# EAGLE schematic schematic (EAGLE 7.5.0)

## Sheet 1 of 3: Supply
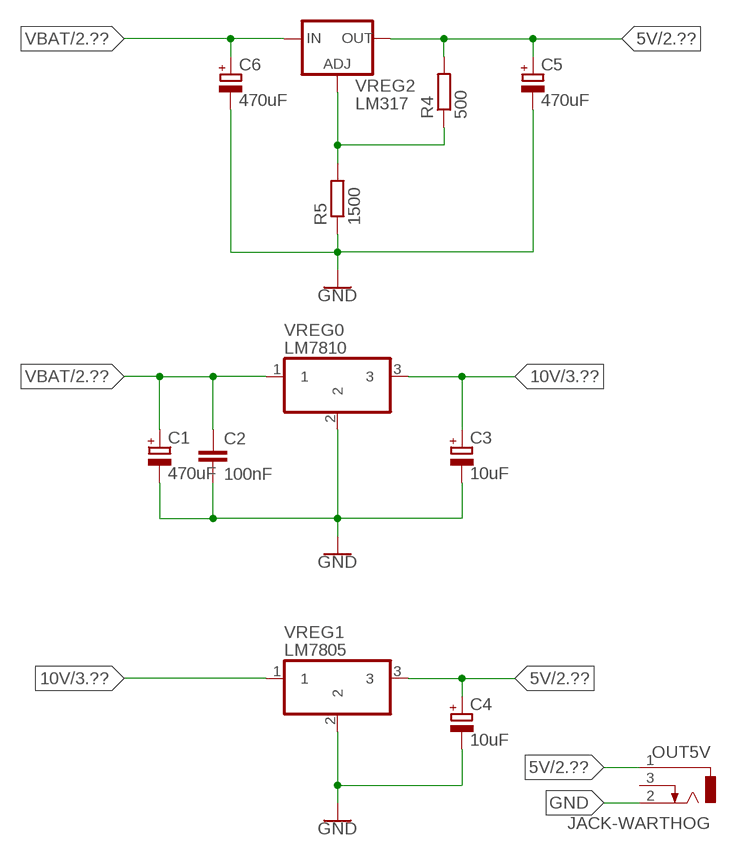
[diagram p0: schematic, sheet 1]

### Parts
C1  470uF  CPOL-EUE3.5-8  [E3,5-8]
C2  100nF  C-EUC0805  [C0805]
C3  10uF  CPOL-EUSMCC  [SMC_C]
C4  10uF  CPOL-EUSMCC  [SMC_C]
C5  470uF  CPOL-EUSMCC  [SMC_C]
C6  470uF  CPOL-EUSMCC  [SMC_C]
OUT5V  JACK-WARTHOG  [JACK-WARTHOG]
R4  500  R-EU_R0805  [R0805]
R5  1500  R-EU_R0805  [R0805]
VREG0  LM7810  TO220V-WARTHOG  [TO220V-WARTHOG]
VREG1  LM7805  TO220V-WARTHOG  [TO220V-WARTHOG]
VREG2  LM317  V_REG_317DPACK  [V-REG_DPACK]

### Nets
5V: C4.+ C5.+ OUT5V.1 R4.2 VREG1.3 VREG2.4(OUT) ; also sheet 2,3
10V: C3.+ VREG0.3 VREG1.1 ; also sheet 3
ADJ: R4.1 R5.2 VREG2.1(ADJ)
GND: C1.- C2.2 C3.- C4.- C5.- C6.- OUT5V.2 R5.1 VREG0.2 VREG1.2 ; also sheet 2,3
VBAT: C1.+ C2.1 C6.+ VREG0.1 VREG2.3(IN) ; also sheet 2,3
Unconnected: OUT5V.3

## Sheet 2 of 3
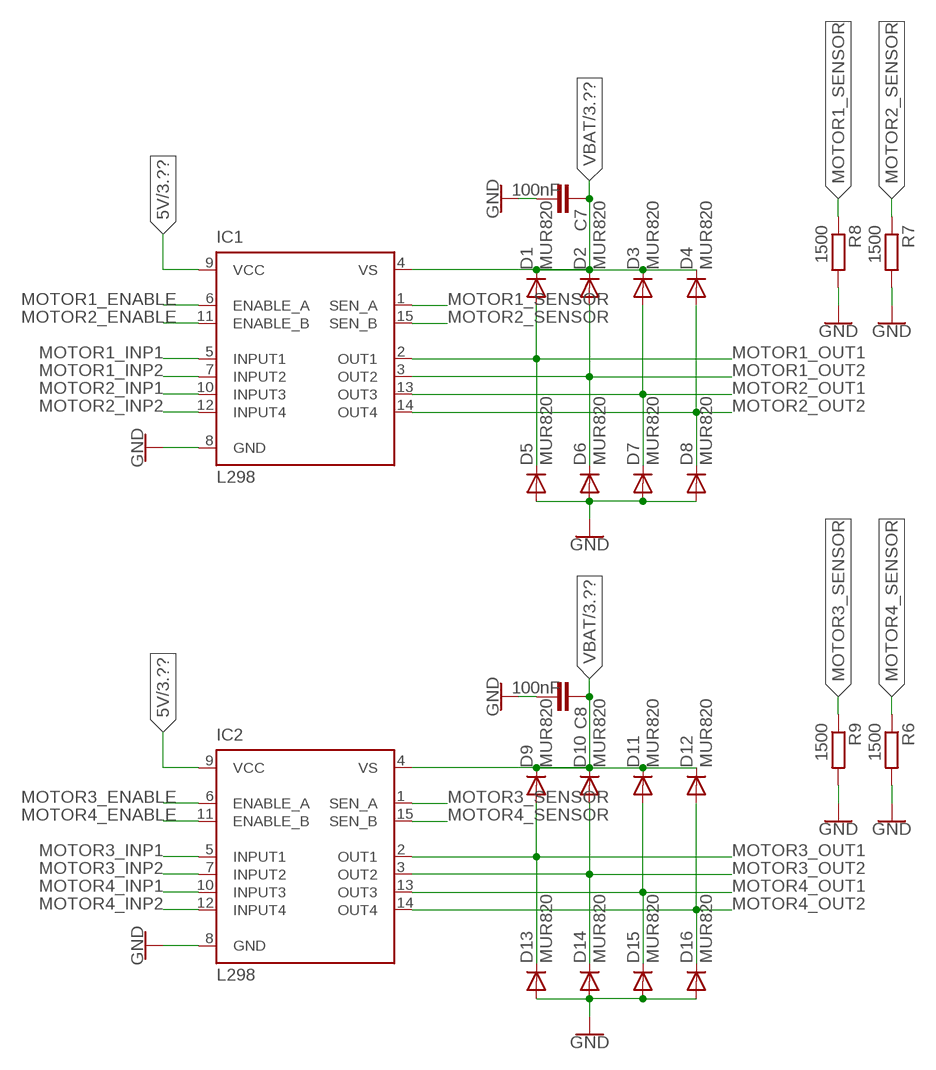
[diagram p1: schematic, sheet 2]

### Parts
C7  100nF  C-EUC0805  [C0805]
C8  100nF  C-EUC0805  [C0805]
D1  MUR820  [C221B1A]
D2  MUR820  [C221B1A]
D3  MUR820  [C221B1A]
D4  MUR820  [C221B1A]
D5  MUR820  [C221B1A]
D6  MUR820  [C221B1A]
D7  MUR820  [C221B1A]
D8  MUR820  [C221B1A]
D9  MUR820  [C221B1A]
D10  MUR820  [C221B1A]
D11  MUR820  [C221B1A]
D12  MUR820  [C221B1A]
D13  MUR820  [C221B1A]
D14  MUR820  [C221B1A]
D15  MUR820  [C221B1A]
D16  MUR820  [C221B1A]
IC1  L298  [MULTIWATT-15]
IC2  L298  [MULTIWATT-15]
R6  1500  R-EU_R0805  [R0805]
R7  1500  R-EU_R0805  [R0805]
R8  1500  R-EU_R0805  [R0805]
R9  1500  R-EU_R0805  [R0805]

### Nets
5V: IC1.9(VCC) IC2.9(VCC) ; also sheet 1,3
GND: C7.2 C8.2 D5.A D6.A D7.A D8.A D13.A D14.A D15.A D16.A IC1.8(GND) IC2.8(GND) R6.2 R7.2 R8.2 R9.2 ; also sheet 1,3
MOTOR1_ENABLE: IC1.6(ENABLE_A)
MOTOR1_INP1: IC1.5(INPUT1)
MOTOR1_INP2: IC1.7(INPUT2)
MOTOR1_OUT1: D1.A D5.C IC1.2(OUT1)
MOTOR1_OUT2: D2.A D6.C IC1.3(OUT2)
MOTOR1_SENSOR: IC1.1(SEN_A) R8.1
MOTOR2_ENABLE: IC1.11(ENABLE_B)
MOTOR2_INP1: IC1.10(INPUT3)
MOTOR2_INP2: IC1.12(INPUT4)
MOTOR2_OUT1: D3.A D7.C IC1.13(OUT3)
MOTOR2_OUT2: D4.A D8.C IC1.14(OUT4)
MOTOR2_SENSOR: IC1.15(SEN_B) R7.1
MOTOR3_ENABLE: IC2.6(ENABLE_A)
MOTOR3_INP1: IC2.5(INPUT1)
MOTOR3_INP2: IC2.7(INPUT2)
MOTOR3_OUT1: D9.A D13.C IC2.2(OUT1)
MOTOR3_OUT2: D10.A D14.C IC2.3(OUT2)
MOTOR3_SENSOR: IC2.1(SEN_A) R9.1
MOTOR4_ENABLE: IC2.11(ENABLE_B)
MOTOR4_INP1: IC2.10(INPUT3)
MOTOR4_INP2: IC2.12(INPUT4)
MOTOR4_OUT1: D11.A D15.C IC2.13(OUT3)
MOTOR4_OUT2: D12.A D16.C IC2.14(OUT4)
MOTOR4_SENSOR: IC2.15(SEN_B) R6.1
VBAT: C7.1 C8.1 D1.C D2.C D3.C D4.C D9.C D10.C D11.C D12.C IC1.4(VS) IC2.4(VS) ; also sheet 1,3

## Sheet 3 of 3: Debug
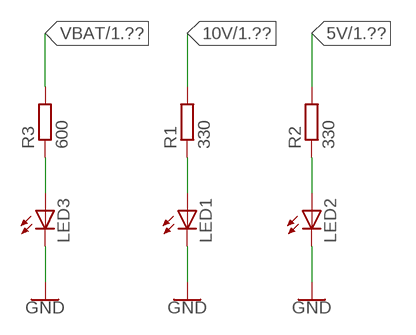
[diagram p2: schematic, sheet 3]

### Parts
LED1  LEDCHIP-LED0805  [CHIP-LED0805]
LED2  LEDCHIP-LED0805  [CHIP-LED0805]
LED3  LEDCHIP-LED0805  [CHIP-LED0805]
R1  330  R-EU_R0805  [R0805]
R2  330  R-EU_R0805  [R0805]
R3  600  R-EU_R0805  [R0805]

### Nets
5V: R2.2 ; also sheet 1,2
10V: R1.2 ; also sheet 1
GND: LED1.C LED2.C LED3.C ; also sheet 1,2
N$1: LED1.A R1.1
N$2: LED2.A R2.1
N$3: LED3.A R3.1
VBAT: R3.2 ; also sheet 1,2

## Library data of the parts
C1 C3-C6 = rcl:CPOL-EU: POLARIZED CAPACITOR, European symbol
C2 C7 C8 = rcl:C-EU: CAPACITOR, European symbol
D1-D16 = diode:MUR820: DIODE
IC1 IC2 = st-microelectronics:L298: DUAL FULL-BRIDGE DRIVER; MPN: L298N; OC_FARNELL: 1589425; OC_NEWARK: 32M1527
LED1-LED3 = adafruit_arduino:LED: LED
OUT5V = JACK-WARTHOG:JACK-WARTHOG
R1-R9 = rcl:R-EU_: RESISTOR, European symbol
VREG0 VREG1 = TO220V-WARTHOG:TO220V-WARTHOG
VREG2 = SparkFun-IC-Power:V_REG_317: Voltage Regulator Standard LM317 adjustable voltage regulator. AOI (Adjust Output Input). Google 'LM317 Calculator' for easy to use app to get the two resistor values needed. 240/720 for 5V output. 240/390 for 3.3V output. Spark Fun Electronics SKU : COM-00527; PROD_ID: IC-09888

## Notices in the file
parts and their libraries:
SparkFun-PowerSymbols: Licensing: Creative Commons ShareAlike 4.0 International - https://creativecommons.org/licenses/by-sa/4.0
